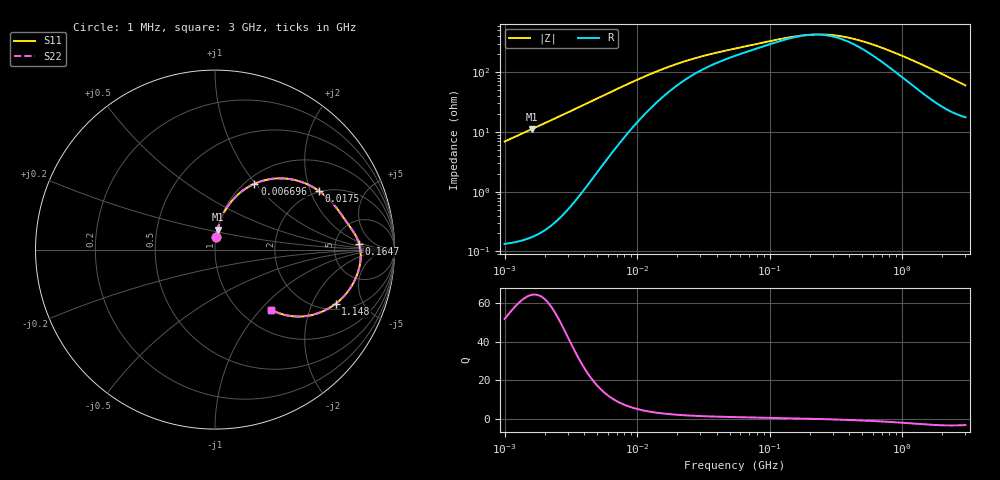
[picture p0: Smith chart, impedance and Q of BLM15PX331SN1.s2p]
! BLM15PX331SN1
# Hz S RI R 50
!Freq.(Hz) S11(Real) S11(Imag) S21(Real) S21(Imag) S12(Real) S12(Imag) S22(Real) S22(Imag)
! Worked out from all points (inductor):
!   401 points, 1 MHz to 3 GHz, reference 50 ohm
!   read as one part in series: L = 1.1 uH near 1.041 MHz
!   highest Q = 64.3 at 1.617 MHz (marker M1), where L = 1.11 uH
!   self-resonance near 209.2 MHz
!   S11 on the Smith chart (normalised r, x): 1 MHz: 1.00, +0.14; 6.696 MHz: 1.10, +0.99; 17.5 MHz: 1.95, +2.29; 164.7 MHz: 8.95, +1.50; 1.148 GHz: 2.30, -3.03; 3 GHz: 1.35, -1.15
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1000000  0.00609 0.0687  0.9939 -0.0687  0.9939 -0.0687  0.00609 0.0687
1616692  0.0142 0.1107  0.9858 -0.1107  0.9858 -0.1107  0.0142 0.1107
2613693  0.0361 0.1768  0.9639 -0.1768  0.9639 -0.1768  0.0361 0.1768
3823119  0.0774 0.2502  0.9226 -0.2502  0.9226 -0.2502  0.0774 0.2502
5059610  0.1337 0.3118  0.8663 -0.3118  0.8663 -0.3118  0.1337 0.3118
6696013  0.2195 0.3666  0.7805 -0.3666  0.7805 -0.3666  0.2195 0.3666
9794439  0.372 0.3971  0.628 -0.3971  0.628 -0.3971  0.372 0.3971
1.461624e7  0.5246 0.3593  0.4754 -0.3593  0.4754 -0.3593  0.5246 0.3593
1.750132e7  0.5778 0.3279  0.4222 -0.3279  0.4222 -0.3279  0.5778 0.3279
2.773354e7  0.6685 0.2428  0.3315 -0.2428  0.3315 -0.2428  0.6685 0.2428
5.477226e7  0.7369 0.1488  0.2631 -0.1488  0.2631 -0.1488  0.7369 0.1488
1.646891e8  0.8035 0.0297  0.1965 -0.0297  0.1965 -0.0297  0.8035 0.0297
2.094008e8  0.8096 -0.000138  0.1904 0.000138  0.1904 0.000138  0.8096 -0.000138
2.827291e8  0.8118 -0.0404  0.1882 0.0404  0.1882 0.0404  0.8118 -0.0404
3.817355e8  0.8069 -0.0854  0.1931 0.0854  0.1931 0.0854  0.8069 -0.0854
5.258324e8  0.7916 -0.1403  0.2084 0.1403  0.2084 0.1403  0.7916 -0.1403
8.005644e8  0.7465 -0.225  0.2535 0.225  0.2535 0.225  0.7465 -0.225
1.147801e9  0.6714 -0.3023  0.3286 0.3023  0.3286 0.3023  0.6714 -0.3023
1.519029e9  0.5824 -0.3515  0.4176 0.3515  0.4176 0.3515  0.5824 -0.3515
1.893158e9  0.4961 -0.3715  0.5039 0.3715  0.5039 0.3715  0.4961 -0.3715
2.359433e9  0.4048 -0.3674  0.5952 0.3674  0.5952 0.3674  0.4048 -0.3674
3e9  0.3144 -0.3355  0.6856 0.3355  0.6856 0.3355  0.3144 -0.3355
